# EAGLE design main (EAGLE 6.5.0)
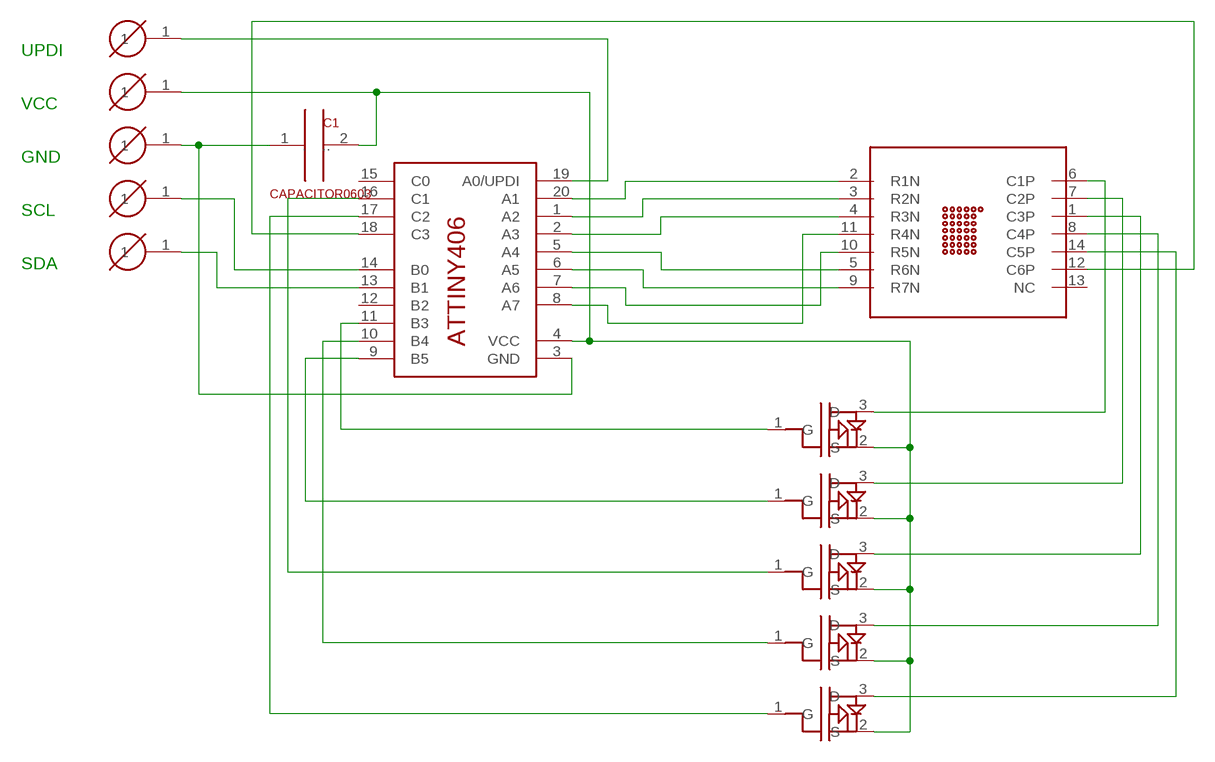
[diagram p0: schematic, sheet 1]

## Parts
C1  CAPACITOR0603  [0603]
DISP  3LS363A  [RUSSIAN_DIP_14]
P_GND  PTH_PIN  [PTH_PIN]
P_SCL  PTH_PIN  [PTH_PIN]
P_SDA  PTH_PIN  [PTH_PIN]
P_UPDI  PTH_PIN  [PTH_PIN]
P_VCC  PTH_PIN  [PTH_PIN]
Q1  PMV50UPE  [SOT23-3]
Q2  PMV50UPE  [SOT23-3]
Q3  PMV50UPE  [SOT23-3]
Q4  PMV50UPE  [SOT23-3]
Q5  PMV50UPE  [SOT23-3]
U1  ATTINY406  [VQFN20]

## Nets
ADC1: DISP.6(C1P) Q1.3(D)
ADC2: DISP.7(C2P) Q2.3(D)
ADC3: DISP.1(C3P) Q3.3(D)
ADC4: DISP.8(C4P) Q4.3(D)
ADC5: DISP.14(C5P) Q5.3(D)
DC1: Q1.1(G) U1.11(B3)
DC2: Q2.1(G) U1.9(B5)
DC3: Q3.1(G) U1.16(C1)
DC4: Q4.1(G) U1.10(B4)
DC5: Q5.1(G) U1.17(C2)
DC6: DISP.12(C6P) U1.18(C3)
DR1: DISP.2(R1N) U1.20(A1)
DR2: DISP.3(R2N) U1.1(A2)
DR3: DISP.4(R3N) U1.2(A3)
DR4: DISP.11(R4N) U1.8(A7)
DR5: DISP.10(R5N) U1.7(A6)
DR6: DISP.5(R6N) U1.5(A4)
DR7: DISP.9(R7N) U1.6(A5)
GND: C1.1(..) P_GND.1 U1.3(GND)
SCL: P_SCL.1 U1.14(B0)
SDA: P_SDA.1 U1.13(B1)
UPDI: P_UPDI.1 U1.19(A0/UPDI)
VCC: C1.2(.) P_VCC.1 Q1.2(S) Q2.2(S) Q3.2(S) Q4.2(S) Q5.2(S) U1.4(VCC)
Unconnected: DISP.13(NC) U1.12(B2) U1.15(C0)

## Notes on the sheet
- UPDI
- VCC
- GND
- SCL
- SDA

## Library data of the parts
C1 = dmitrygr:CAPACITOR
DISP = dmitrygr:3LS363A
P_GND P_SCL P_SDA P_UPDI P_VCC = dmitrygr:PTH_PIN
Q1-Q5 = dmitrygr:PMV50UPE
U1 = dmitrygr:ATTINY406

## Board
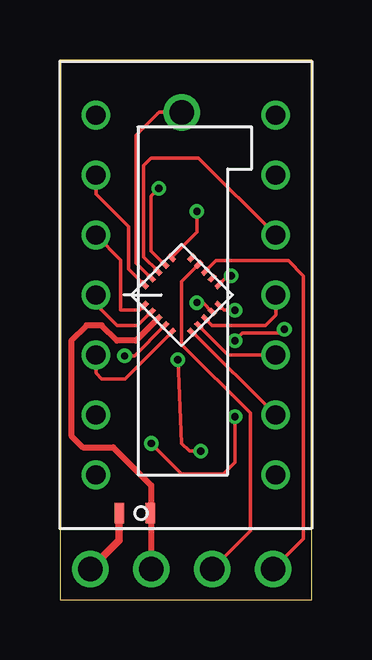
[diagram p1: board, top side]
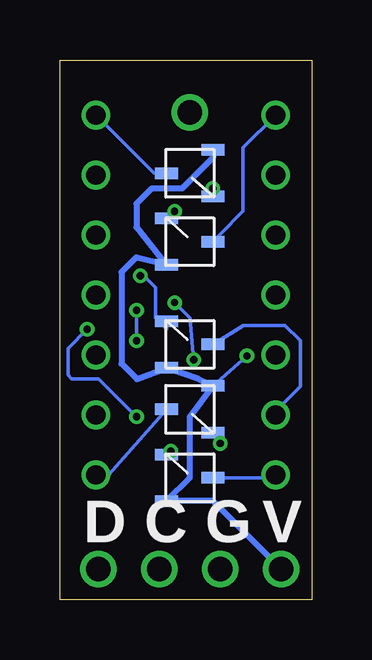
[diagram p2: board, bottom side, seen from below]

Size 10.5 x 22.5 mm. Coordinates in mm from the lower left corner, seen from the top.
Outline: 0,0 10.5,0 10.5,22.5 0,22.5 0,0
Copper layers (1*16): Top 0.035mm / dielectric 1.5mm / Bottom 0.035mm
Design rules "MF_Standard_2_Layer": minimum track width 5mil, minimum drill 12mil, track to track 5mil, track to pad 5mil, pad to pad 5mil, via to via 5mil, smd to smd 0mil, copper to edge 10mil, drill to drill 10mil, minimum pad ring 6mil, minimum via ring 6mil, stop-mask expansion 2mil, vias tented up to drill 25mil, thermal gap 10mil

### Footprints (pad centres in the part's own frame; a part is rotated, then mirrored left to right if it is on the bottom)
0603 = smd 0.4 x 0.85: 1 -0.65,0; 2 0.65,0
RUSSIAN_DIP_14 = drill 0.8: 1 -3.75,7.5; 2 -3.75,5; 3 -3.75,2.5; 4 -3.75,0; 5 -3.75,-2.5; 6 -3.75,-5; 7 -3.75,-7.5; 8 3.75,-7.5; 9 3.75,-5; 10 3.75,-2.5; 11 3.75,0; 12 3.75,2.5; 13 3.75,5; 14 3.75,7.5
PTH_PIN = drill 1.016: 1 0,0
SOT23-3 = smd 0.48 x 0.95: 1 0.97,0.97; 2 -0.97,0.97; 3 0,-0.97
VQFN20 = smd 0.35 x 0.2: 1 -1.4,0.8; 2 -1.4,0.4; 3 -1.4,0; 4 -1.4,-0.4; 5 -1.4,-0.8; 11 1.4,-0.8; 12 1.4,-0.4; 13 1.4,0; 14 1.4,0.4; 15 1.4,0.8 | smd 0.2 x 0.35: 6 -0.8,-1.4; 7 -0.4,-1.4; 8 0,-1.4; 9 0.4,-1.4; 10 0.8,-1.4; 16 0.8,1.4; 17 0.4,1.4; 18 0,1.4; 19 -0.4,1.4; 20 -0.8,1.4

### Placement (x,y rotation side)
C1  3.13,3.6 180 top
DISP  5.25,12.7 0 top
P_GND  3.81,1.27 0 top
P_SCL  6.35,1.27 0 top
P_SDA  8.89,1.27 0 top
P_UPDI  5.08,20.32 0 top
P_VCC  1.27,1.27 0 top
Q1  5.08,10.64 90 bottom
Q2  5.08,5.08 90 bottom
Q3  5.08,14.92 90 bottom
Q4  5.08,7.94 270 bottom
Q5  5.08,17.78 270 bottom
U1  5.08,12.7 45 top

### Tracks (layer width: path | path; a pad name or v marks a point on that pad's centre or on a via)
ADC1
  Bottom 0.152: Q1.3 2.84,11.43 1.11,11.43 0.48,10.79 0.48,8.89 1.5,7.87 DISP.6
ADC2
  Bottom 0.152: Q2.3 1.5,5.08 DISP.7
ADC3
  Bottom 0.152: Q3.3 3.81,15.24 2.86,16.19 2.86,18.84 DISP.1
ADC4
  Bottom 0.152: DISP.8 8.47,5.2 Q4.3
ADC5
  Bottom 0.152: Q5.3 6.58,17.78 DISP.14
DC1  (via drill 0.3)
  Top 0.152: U1.11 6.64,13.14 6.99,13.49 v7.14,13.49
  Bottom 0.152: Q1.1 6.05,11.29 6.51,11.75 6.51,13.02 6.99,13.49 v7.14,13.49
DC2  (via drill 0.3)
  Top 0.152: U1.9 5.96,12.38 v5.71,12.38 | v4.92,10 5.08,6.51 5.4,6.19 v5.87,6.19
  Bottom 0.152: v5.71,12.38 5.08,11.75 v4.92,10 | Q2.1 5.91,6.19 v5.87,6.19
DC3  (via drill 0.3)
  Top 0.152: v5.71,16.19 5.71,15.31 U1.16
  Bottom 0.152: Q3.1 5.73,16.21 v5.71,16.19
DC4  (via drill 0.3)
  Top 0.152: U1.10 6.85,12.06 v7.3,12.06 | v7.3,10.79 7.62,11.11 9.21,11.11 v9.37,11.27 | v3.81,6.51 5.08,5.24 6.83,5.24 7.3,5.71 v7.3,7.62
  Bottom 0.152: v7.3,12.06 v7.3,10.79 | v9.37,11.27 10.16,10.48 10.16,9.37 10,9.21 8.89,9.21 v7.3,7.62 | Q4.1 v3.81,6.51
DC5  (via drill 0.3)
  Top 0.152: v4.13,17.14 3.81,16.83 3.81,14.54 U1.17
  Bottom 0.152: Q5.1 4.13,16.83 v4.13,17.14
DC6
  Top 0.152: U1.18 | U1.18 3.49,14.29 3.49,18.1 3.81,18.41 5.79,18.41 DISP.12
DR1
  Top 0.152: U1.20 2.86,13.79 2.86,15.56 1.5,16.91 DISP.2
DR2
  Top 0.152: U1.1 3.31,12.06 2.54,12.06 2.54,14.16 DISP.3
DR3
  Top 0.152: U1.2 3.24,11.43 2.38,11.43 1.5,12.31 DISP.4
DR4
  Top 0.152: U1.8 6.35,11.43 8.57,11.43 9,11.86 DISP.11
DR5
  Top 0.152: U1.7 7.01,10.2 DISP.10
DR6
  Top 0.152: U1.5 2.72,9.21 1.75,9.21 1.5,9.45 DISP.5
DR7
  Top 0.152: U1.6 5.56,11.14 DISP.9
GND
  Top 0.254: U1.3 3.17,10.79 2.38,10.79 1.75,11.43 1.11,11.43 0.48,10.79 0.48,6.83 0.95,6.35 2.22,6.35 3.81,4.76 3.81,3.65 P_GND.1
  Top 0.305: C1.1 3.81,3.64 3.81,3.65
SCL
  Top 0.152: U1.14 5.08,13.27 5.08,10.64 7.94,7.78 7.94,2.86 P_SCL.1
SDA
  Top 0.152: U1.13 6.51,14.13 9.53,14.13 10.16,13.49 10.16,2.54 P_SDA.1
UPDI
  Top 0.152: U1.19 3.17,14.04 3.17,19.37 4.13,20.32 P_UPDI.1
VCC  (via drill 0.3)
  Top 0.152: U1.4 3.11,10.16 v2.7,10.16
  Top 0.305: P_VCC.1 2.48,2.48 C1.2
  Bottom 0.152: v2.7,10.16 Q4.2
  Bottom 0.254: Q5.2 4.11,18.43 5.4,17.14 6.67,17.14 7.3,16.51 7.3,15.52 Q3.2 7.32,14.27 7.94,13.65 7.94,9.84 7.29,9.19 Q1.2 4.71,9.19 Q4.2 5.08,7.62 5.08,5.08 Q2.2 4.11,4.11 P_VCC.1

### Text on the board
bPlace: V | G | C | D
